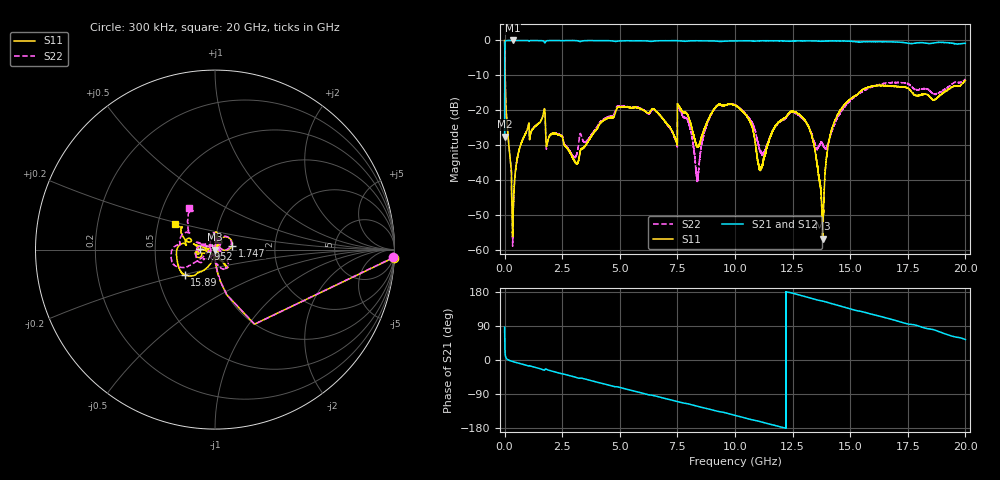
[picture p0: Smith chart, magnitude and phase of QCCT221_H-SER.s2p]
! Created Fri Feb  5 15:38:22 2021
# hz S ma R 50
! 2 Port Network Data from SP1.SP block
! freq  magS11  angS11  magS21  angS21  magS12  angS12  magS22  angS22
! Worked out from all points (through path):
!   20001 points, 300 kHz to 20 GHz, reference 50 ohm
!   highest |S21| = -0.01 dB at 345.3 MHz (marker M1); lowest = -27.5 dB at 300 kHz (marker M2)
!   group delay of S21, straight-line fit = 42.3 ps
!   lowest |S11| = -56.8 dB at 13.8 GHz (marker M3), VSWR 1.00, Z = 49.9 - j0.00555 ohm
!   |S11| at or under -10 dB: 21.21 MHz to end of sweep
!   |S22| runs from -58.9 to -0.1 dB; largest |S21 - S12| = 0.014
!   S11 on the Smith chart (normalised r, x): 300 kHz: 4, -44; 1.747 GHz: 1.21, +0.06; 7.952 GHz: 0.84, +0.00; 15.89 GHz: 0.69, -0.20; 20 GHz: 0.61, +0.19
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300000  0.9963 -2.6  0.04206 86.9  0.04224 87.6  0.9935 -2.5
1.033e8  0.06455 -88.4  0.9968 2.4  0.997 2.4  0.06499 -88.5
3.453e8  0.001655 -162.6  0.9991 -3.9  0.9978 -3.9  0.001446 -156.0
9.643e8  0.05059 77.1  0.9982 -14.2  0.998 -14.2  0.05074 75.9
1.7473e9  0.09814 13.4  0.9234 -25.7  0.9232 -25.7  0.09534 16.0
3.3343e9  0.02827 -110.8  0.9752 -47.7  0.9755 -47.7  0.04299 -84.0
4.9573e9  0.1118 -162.7  0.9812 -71.7  0.9807 -71.6  0.1153 -149.3
6.6673e9  0.09046 -178.4  0.9882 -96.8  0.9882 -96.8  0.0899 169.0
7.3993e9  0.04005 175.1  0.9919 -108.1  0.9923 -108.1  0.03868 155.1
7.6003e9  0.1109 167.7  0.9833 -111.2  0.9847 -111.2  0.1023 156.9
7.9523e9  0.08491 179.0  0.979 -115.5  0.9797 -115.4  0.07016 154.3
8.3683e9  0.0304 -127.8  0.9894 -122.1  0.9895 -122.0  0.009923 52.7
9.0103e9  0.09429 -57.5  0.9821 -131.8  0.9829 -131.7  0.09236 -42.2
1.00003e10  0.1179 -55.3  0.9828 -146.0  0.9837 -146.1  0.1193 -66.2
1.10973e10  0.01402 -0.1  0.9878 -162.7  0.9859 -162.7  0.02615 -157.0
1.24153e10  0.09541 88.9  0.9748 177.6  0.9734 177.4  0.0934 101.5
1.33343e10  0.04336 74.2  0.9871 162.6  0.9855 162.5  0.04542 88.1
1.38023e10  0.00145 -177.8  0.9735 155.3  0.9723 155.4  0.03238 144.8
1.43453e10  0.07157 -105.8  0.9805 146.3  0.9828 146.2  0.06538 -150.3
1.58903e10  0.2188 -140.2  0.9602 121.5  0.9632 121.6  0.2133 -152.2
1.66673e10  0.2225 -156.3  0.9545 109.2  0.9454 109.0  0.2465 -161.0
2e10  0.2676 147.4  0.9091 54.0  0.9006 53.7  0.2786 122.0
